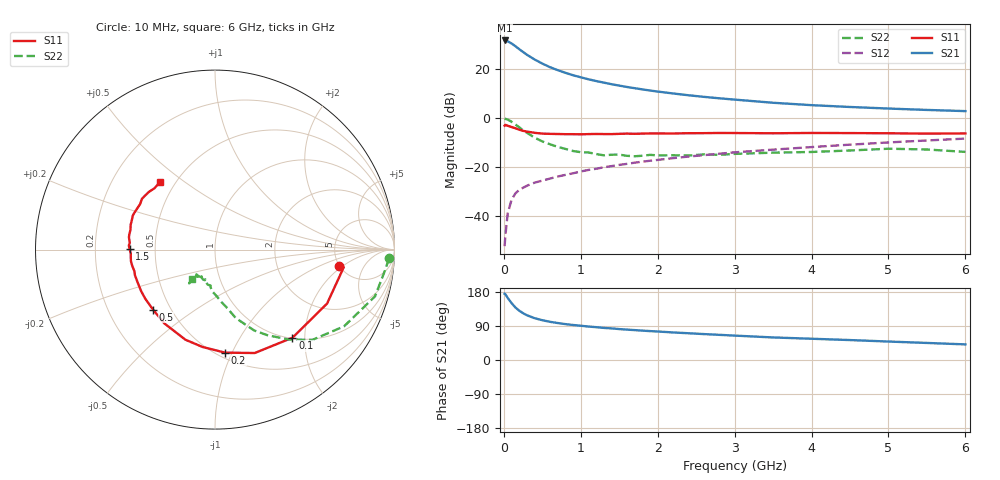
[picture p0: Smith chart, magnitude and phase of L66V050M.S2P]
!  INFINEON TECHNOLOGIES Small Signal Semiconductors
! BFR380L3 , Si-NPN RF-Transistor in TSLP-3-1
!  Vce=6 V,  Ic=50 mA
! Common Emitter S-Parameters:  07. March 2005
#  GHz  S  MA  R  50
! f  S11  S21  S12  S22
! GHz  Mag  Ang  Mag  Ang  Mag  Ang  Mag  Ang
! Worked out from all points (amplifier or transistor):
!   36 points, 10 MHz to 6 GHz, reference 50 ohm
!   highest |S21| = 31.4 dB at 10 MHz (marker M1)
!   |S21| within 3 dB of that: start of sweep to 178.3 MHz
!   unconditionally stable (mu >= 1): 1.812 GHz to 4.779 GHz
!   at 250 MHz: K = 0.43, MSG = 27.6 dB, |S12| = -28.3 dB
!   at 1.4 GHz: K = 0.97, MSG = 16.6 dB, |S12| = -19.6 dB
!   at 6 GHz: K = 0.97, MSG = 5.6 dB, |S12| = -8.4 dB
!   S11 on the Smith chart (normalised r, x): 10 MHz: 4.96, -1.79; 100 MHz: 1.01, -1.74; 200 MHz: 0.55, -0.94; 500 MHz: 0.40, -0.35; 1.5 GHz: 0.36, +0.00; 6 GHz: 0.41, +0.40
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0.01  0.6983 -7.6  37.33 174.7  0.0025 64.4  0.9706 -2.9
0.02  0.7241 -7.8  36.98 173.5  0.0041 83.9  0.9562 -6.5
0.05  0.6931 -25.7  35.88 163.9  0.0115 76.4  0.9288 -16.3
0.1  0.6537 -48.7  32.43 150.2  0.0218 68.8  0.8367 -30.7
0.15  0.6172 -69.0  28.6 138.7  0.0294 62.3  0.7395 -42.9
0.2  0.5769 -84.4  24.87 130.1  0.0347 58.8  0.6458 -50.8
0.25  0.5467 -97.4  21.8 123.5  0.0383 56.1  0.5595 -58.5
0.3  0.5284 -108.2  19.14 118.1  0.0421 54.8  0.5 -64.2
0.4  0.4986 -124.6  15.34 110.3  0.0486 54.2  0.3977 -73.2
0.5  0.4805 -136.0  12.67 105.0  0.0535 55.3  0.3338 -78.1
0.6  0.4753 -144.7  10.72 100.8  0.0588 56.4  0.2924 -83.3
0.8  0.4682 -157.1  8.233 94.7  0.0699 59.1  0.2354 -93.2
0.9  0.4683 -162.3  7.347 92.4  0.0753 60.4  0.2131 -96.5
1.1  0.47 -168.9  6.088 88.3  0.0881 62.3  0.1991 -101.9
1.5  0.4755 179.8  4.527 81.6  0.1114 64.3  0.1801 -111.4
1.8  0.4806 173.4  3.797 77.5  0.1295 65.3  0.1708 -116.7
2.2  0.4837 166.9  3.135 72.7  0.1529 65.4  0.1748 -120.5
2.8  0.4955 157.6  2.503 66.4  0.1878 65.6  0.1783 -127.7
3.5  0.4884 148.7  2.031 59.5  0.2273 63.8  0.1975 -127.3
4.5  0.4928 142.8  1.668 52.6  0.2869 62.5  0.2186 -127.4
5.5  0.4801 134.6  1.453 45.0  0.3489 59.0  0.2289 -127.1
6  0.4851 129.5  1.375 41.2  0.381 57.0  0.2045 -127.9
